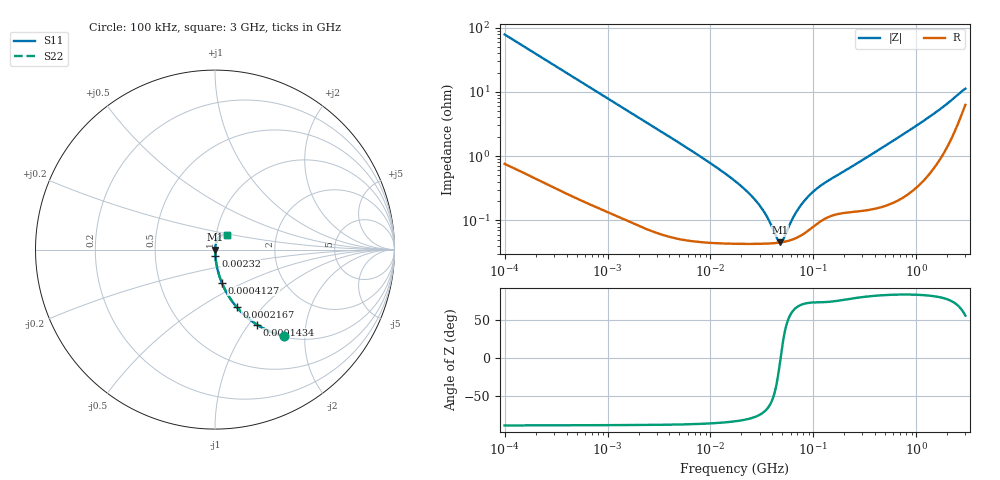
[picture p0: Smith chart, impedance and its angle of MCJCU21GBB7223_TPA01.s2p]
! MCJCU21GBB7223_TPA01  S-PARAMETER MODEL  ( Standard Model )
! Model Generated by TAIYO YUDEN Corporation (http://www.ty-top.com)
! Version 1.0
! TAIYO YUDEN Control No. 220601
! Copyright(c) 2015 TAIYO YUDEN CO.,LTD. All Rights Reserved.
! Product Description (link to TY-COMPAS)
! https://ds.yuden.co.jp/TYCOMPAS/or/detail?pn=MCJCU21GBB7223KTPA01&u=M
! Products Name : Multilayer Ceramic Capacitors
! Characteristics :
!  Capacitance : 0.022 [uF] , Rated Voltage : 50 [V] , TCC : X7R
!  Case Size : 2.0 x 1.25 / 0.079 x 0.049 [mm/inch] , Thickness : 1.25 / 0.049 [mm/inch]
!  (Conditions: Temperature = 25 [degC] , DC Bias Voltage = 0 [V])
! External Node Assignments :
!  1  o---| |---o  2
! GND o---------o GND
! Frequency Range : 100kHz  -  3GHz  [ 401 STEP ]
# MHZ S RI R 50
! Freq[MHz].  S11 Real  S11 Imag  S21 Real  S21 Imag  S12 Real  S12 Imag  S22 Real  S22 Imag
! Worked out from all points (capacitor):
!   401 points, 100 kHz to 3 GHz, reference 50 ohm
!   read as one part in series: C = 20.2 nF near 105.3 kHz
!   lowest |Z| = 45.4 mohm at 47.32 MHz (marker M1)
!   series resonance near 48.03 MHz, so ESL is about 540 pH
!   S11 on the Smith chart (normalised r, x): 100 kHz: 1.02, -1.57; 143.4 kHz: 1.01, -1.10; 216.7 kHz: 1.01, -0.73; 412.7 kHz: 1.01, -0.38; 2.32 MHz: 1.00, -0.07; 3 GHz: 1.13, +0.19
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0.1  0.3823 -0.4812  0.6177 0.4812  0.6177 0.4812  0.3823 -0.4812
0.14345  0.2336 -0.4179  0.7664 0.4179  0.7664 0.4179  0.2336 -0.4179
0.216663  0.1199 -0.3191  0.8801 0.3191  0.8801 0.3191  0.1199 -0.3191
0.412671  0.0378 -0.1843  0.9622 0.1843  0.9622 0.1843  0.0378 -0.1843
0.562235  0.0215 -0.138  0.9785 0.138  0.9785 0.138  0.0215 -0.138
2.320182  0.00194 -0.0345  0.9981 0.0345  0.9981 0.0345  0.00194 -0.0345
3.161081  0.00126 -0.0253  0.9987 0.0253  0.9987 0.0253  0.00126 -0.0253
9.574722  0.000512 -0.0081  0.9995 0.0081  0.9995 0.0081  0.000512 -0.0081
17.7727  0.000445 -0.00393  0.9996 0.00393  0.9996 0.00393  0.000445 -0.00393
24.21403  0.000435 -0.0025  0.9996 0.0025  0.9996 0.0025  0.000435 -0.0025
30.53531  0.000433 -0.00159  0.9996 0.00159  0.9996 0.00159  0.000433 -0.00159
36.57227  0.000435 -0.000939  0.9996 0.000939  0.9996 0.000939  0.000435 -0.000939
44.94634  0.000446 -0.000227  0.9996 0.000227  0.9996 0.000227  0.000446 -0.000227
47.32384  0.000451 -5.02e-05  0.9995 5.02e-05  0.9995 5.02e-05  0.000451 -5.02e-05
51.12795  0.00046 0.000215  0.9995 -0.000215  0.9995 -0.000215  0.00046 0.000215
62.83488  0.000503 0.000937  0.9995 -0.000937  0.9995 -0.000937  0.000503 0.000937
71.47675  0.000552 0.00141  0.9994 -0.00141  0.9994 -0.00141  0.000552 0.00141
97.38194  0.000775 0.00259  0.9992 -0.00259  0.9992 -0.00259  0.000775 0.00259
132.6759  0.00109 0.00379  0.9989 -0.00379  0.9989 -0.00379  0.00109 0.00379
547.5153  0.00201 0.0158  0.998 -0.0158  0.998 -0.0158  0.00201 0.0158
1838.476  0.0141 0.0567  0.9859 -0.0567  0.9859 -0.0567  0.0141 0.0567
3000  0.0663 0.0819  0.9337 -0.0819  0.9337 -0.0819  0.0663 0.0819
